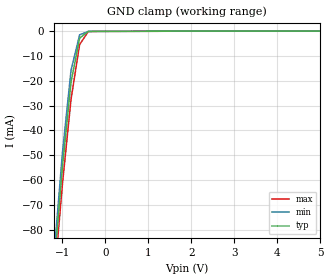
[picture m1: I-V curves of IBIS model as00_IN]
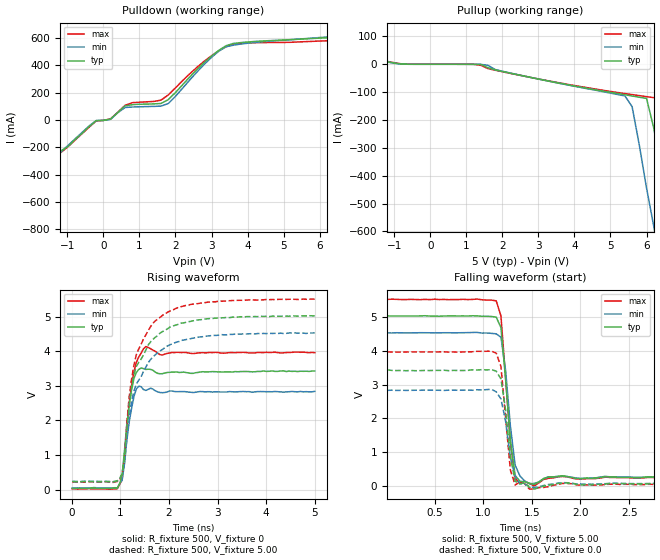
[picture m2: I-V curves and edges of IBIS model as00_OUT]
| TEXas INSTRUMENTS INCORPORATED
| Standard Linear and Logic Group
| IBIS Model of SN74as00
| QUADRUPLE 2-INPUT POSITIVE-NAND GATES
| SOIC 14-pin (D), SOP 14-pin (NS), PDIP 14-pin (N) packages
[IBIS Ver]   3.2
[Comment Char]  |_char
[File Name]   sn74as00.ibs
[File Rev]   3.1 I_die
[Date]   Sept. 29, 2004
[Source]   File originated at Texas Instruments, Inc.
[Notes]   The following is an IBIS list for the as00.
   - FILE REV HISTORY
   - 3.1 Re-Release IBIS file on 10/06/04
   - Power clamp data deleted as there is no power-clamp diode.
   - All test data contained in this file are derived from
   actual measurements.
   - File created by Nobuhisa Ohtsubo, SLL Product Engineering.
[Disclaimer] Property of Texas Instruments Incorporated.  Unauthorized
   reproduction and/or distribution is strictly prohibited.
   This product is protected under copyright law.
   Created 2000, (C) Copyright 2000, Texas Instruments Inc.,
   All Rights Reserved.
   UNLESS THERE IS A SIGNED, WRITTEN AGREEMENT TO THE
   CONTRARY, TEXas INSTRUMENTS () IS PROVIDING THE IBIS
   MODELS  AND WITHOUT ANY WARRANTY, EXPRESSED OR
   IMPLIED.  TI assumes no liability for:
   1) the accuracy of the IBIS models provided to your
   company;
   2) the proper functioning of these IBIS Models in your
   design or for any resulting applications; or
   3) infringement of patents, copyrights or intellectual
   property rights resulting from your use of these IBIS
   models.
   TI provides IBIS Models as a service to our customers.
   You and your company shall not distribute, sell or give
   these models to anyone else without prior written
   permission from TI.
   TI reserves the right to make changes to our products or
   to discontinue any semiconductor product or service
   without notice, and advises our customers to obtain the
   latest version of relevant information to verify, before
   placing orders, that the information being relied on is
   current.
   Please be aware that your receipt and use of the IBIS
   information provided shall serve as acceptance of these
   terms and conditions.  If you do not accept these terms,
   you should return or destroy the IBIS models and any
   other accompanying information immediately.
|   Component as00_D
[Component]   as00_D
[Manufacturer]  Texas Instruments, Inc.
[Package]
|   typ   min   max
R_pkg   0.031   0.028   0.034
L_pkg   3.109nH   2.462nH   3.889nH
C_pkg   0.473pF   0.363pF   0.628pF
[Pin]   signal_name   model_name   R_pin   L_pin   C_pin
1   1A   as00_IN   0.033   3.854nH   0.622pF
2   1B   as00_IN   0.032   3.188nH   0.473pF
3   1Y   as00_OUT   0.028   2.462nH   0.377pF
4   2A   as00_IN   0.031   2.596nH   0.363pF
5   2B   as00_IN   0.028   2.521nH   0.372pF
6   2Y   as00_OUT   0.034   3.250nH   0.476pF
7   GND   GND   0.034   3.889nH   0.628pF
8   3Y   as00_OUT   0.034   3.889nH   0.628pF
9   3A   as00_IN   0.034   3.250nH   0.476pF
10   3B   as00_IN   0.028   2.521nH   0.372pF
11   4Y   as00_OUT   0.031   2.596nH   0.364pF
12   4A   as00_IN   0.028   2.462nH   0.377pF
13   4B   as00_IN   0.032   3.188nH   0.473pF
14   VCC   POWER   0.033   3.854nH   0.622pF
|   Component as00_NS
[Component]   as00_NS
[Manufacturer]  Texas Instruments, Inc.
[Package]
|   typ   min   max
R_pkg   0.045   0.039   0.054
L_pkg   3.796nH   2.561nH   4.952nH
C_pkg   0.528pF   0.288pF   0.710pF
[Pin]   signal_name   model_name   R_pin   L_pin   C_pin
1   1A   as00_IN   0.047   4.867nH   0.706pF
2   1B   as00_IN   0.051   4.083nH   0.592pF
3   1Y   as00_OUT   0.041   2.915nH   0.376pF
4   2A   as00_IN   0.039   2.561nH   0.288pF
5   2B   as00_IN   0.041   3.101nH   0.430pF
6   2Y   as00_OUT   0.047   4.047nH   0.589pF
7   GND   GND   0.051   4.909nH   0.700pF
8   3Y   as00_OUT   0.045   4.784nH   0.694pF
9   3A   as00_IN   0.054   4.176nH   0.597pF
10   3B   as00_IN   0.039   3.287nH   0.449pF
11   4Y   as00_OUT   0.039   2.586nH   0.294pF
12   4A   as00_IN   0.040   2.802nH   0.371pF
13   4B   as00_IN   0.049   4.080nH   0.593pF
14   VCC   POWER   0.052   4.952nH   0.710pF
|   Component as00_N
[Component]   as00_N
[Manufacturer]   Texas Instruments, Inc.
[Package]
|   typ   min   max
R_pkg   4.500e-02   3.700e-02   6.300e-02
L_pkg   5.407e-09   3.922e-09   6.942e-09
C_pkg   3.890e-13   2.050e-13   6.040e-13
[Pin]   signal_name   model_name   R_pin   L_pin   C_pin
1   1A   as00_IN   6.300e-02   6.942e-09   6.040e-13
2   1B   as00_IN   3.700e-02   6.200e-09   4.060e-13
3   1Y   as00_OUT   4.200e-02   4.389e-09   3.220e-13
4   2A   as00_IN   3.800e-02   3.922e-09   2.050e-13
5   2B   as00_IN   3.900e-02   4.301e-09   2.980e-13
6   2Y   as00_OUT   3.800e-02   5.329e-09   3.560e-13
7   GND   GND   5.300e-02   6.510e-09   5.440e-13
8   3Y   as00_OUT   5.300e-02   6.437e-09   5.390e-13
9   3A   as00_IN   3.900e-02   5.352e-09   3.470e-13
10   3B   as00_IN   4.200e-02   4.473e-09   2.970e-13
11   4Y   as00_OUT   4.400e-02   4.326e-09   2.250e-13
12   4A   as00_IN   4.200e-02   4.295e-09   2.800e-13
13   4B   as00_IN   4.200e-02   6.318e-09   4.180e-13
14   VCC   POWER   6.100e-02   6.900e-09   6.030e-13
| Models and submodels in the file (2): as00_IN (Input), as00_OUT (Output)
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|   Model as00_IN
[Model]   as00_IN
Model_type  Input
Polarity   Non-Inverting
Vinl = 0.8
Vinh = 2.0
| variable   typ   min   max
C_comp   1.33pf   1.00pf   1.66pf
[Temperature Range]   25   0   70
[Voltage Range]   5.0   4.5   5.5
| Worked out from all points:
|   GND clamp passes 1 mA (typ) near -0.46 V on its own axis
[GND Clamp]
|   Voltage   I(typ)   I(min)   I(max)
-5V       -1.126A    -1.168A    -1.087A
-1.2V     -96.27mA   -91.36mA   -102.1mA
-1V       -54.78mA   -49.12mA   -61.66mA
-800mV    -20.6mA    -15.82mA   -27.49mA
-600mV    -2.839mA   -1.5mA     -5.406mA
-400mV    -139.7uA   -123.8uA   -215.7uA
5V        170pA      183.6pA    226.4pA
|   Model as00_OUT
[Model]   as00_OUT
Model_type  Output
Polarity   Inverting
Enable   Active-Low
Vmeas = 1.3v
Cref = 0pf
| variable   typ   min   max
C_comp   5.8pf   4.35pf   7.25pf
[Temperature Range]   25   0   70
[Voltage Range]   5.0   4.5   5.5
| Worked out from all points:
|   slope of the pulldown table from 0 to 0.75 V, typ, clamps not added: 6.65 ohm
|   slope of the pullup table from 0 to 0.75 V, typ, clamps not added: 22.6 kohm
|   rising waveform, R_fixture 500, V_fixture 0: 20-80 % time 160ps typ, 152ps min, 176ps max; typ from 0.031 V to 3.43 V
|   falling waveform, R_fixture 500, V_fixture 5.00: 20-80 % time 84.4ps typ, 89.7ps min, 82.1ps max; typ from 5.05 V to 0.24 V
|   rising waveform, R_fixture 500, V_fixture 5.00: 20-80 % time 433ps typ, 469ps min, 411ps max; typ from 0.23 V to 5.02 V
|   falling waveform, R_fixture 500, V_fixture 0.0: 20-80 % time 84.8ps typ, 94.7ps min, 74.7ps max; typ from 3.44 V to 0.043 V
[Pulldown]
|   Voltage   I(typ)   I(min)   I(max)
-5V       -2.513A    -2.408A    -2.451A
-2.2V     -859.8mA   -830.5mA   -846.9mA
-2V       -741.7mA   -717.8mA   -732.3mA
-1.6V     -517mA     -521.7mA   -510.6mA
-1.2V     -227.4mA   -239.2mA   -241.5mA
-200mV    -4.196mA   -3.233mA   -5.919mA
200mV     7.396mA    5.741mA    9.506mA
600mV     103.7mA    92.22mA    108mA
1.8V      149.8mA    121.4mA    184.6mA
2.8V      422.2mA    408.7mA    431.4mA
3.4V      544.1mA    536.6mA    537.1mA
10V       655.6mA    682.5mA    620.9mA
[Pullup]
|   Voltage   II(typ)   I(min)   I(max)
-5V       115.7mA    126.5mA    99.43mA
-1V       4.25mA     3.482mA    5.401mA
1.6V      -12.64mA   -3.784mA   -15.45mA
5.4V      -109.5mA   -113.6mA   -105.2mA
5.6V      -113.9mA   -152.3mA   -108.8mA
6V        -122.7mA   -444.5mA   -116.2mA
6.2V      -228.6mA   -581.2mA   -119.9mA
6.4V      -370.2mA   -720.9mA   -123.6mA
6.6V      -518.5mA   -860.6mA   -180.5mA
6.8V      -643.6mA   -1A        -305.7mA
7.2V      -913.2mA   -1.28A     -569.1mA
10V       -2.801A    -3.236A    -2.375A
[Ramp]
| variable   typ   min   max
dV/dt_r   1.940E+00/1.520E-09  1.600E+00/1.490E-09  2.290E+00/1.710E-09
dV/dt_f   2.880E+00/8.100E-10  2.580E+00/8.400E-10  3.180E+00/7.800E-10
R_load = 500
[Rising Waveform]
R_fixture = 500
V_fixture = 0
C_fixture = 0pf
L_fixture = 0nH
|   Time   V(typ)   V(min)   V(max)
9.766ps   31.22mV    44.19mV    19.5mV
937.5ps   42.63mV    43.72mV    22.32mV
1.035ns   414mV      269mV      280.4mV
1.133ns   1.898V     1.425V     1.782V
1.182ns   2.428V     1.956V     2.505V
1.279ns   3.21V      2.688V     3.405V
1.377ns   3.47V      2.987V     3.827V
1.523ns   3.47V      2.865V     4.131V
1.865ns   3.348V     2.798V     3.888V
5ns       3.427V     2.838V     3.954V
[Falling Waveform]
R_fixture = 500
V_fixture = 5.00
V_fixture_min = 4.50
V_fixture_max = 5.50
C_fixture = 0pf
L_fixture = 0nH
|   Time   V(typ)   V(min)   V(max)
9.766ps   5.047V     4.543V     5.538V
1.133ns   5.012V     4.513V     5.495V
1.182ns   4.699V     4.415V     5.045V
1.23ns    3.153V     3.418V     3.192V
1.279ns   1.337V     1.77V      1.285V
1.328ns   299.7mV    603.1mV    200.4mV
1.377ns   127mV      286.4mV    77mV
1.475ns   69.03mV    50.13mV    59.5mV
1.816ns   289.3mV    283.1mV    269.2mV
5ns       239.7mV    246.5mV    230mV
[Rising Waveform]
R_fixture = 500
V_fixture = 5.00
V_fixture_min = 4.50
V_fixture_max = 5.50
C_fixture = 0pf
L_fixture = 0nH
|   Time   V(typ)   V(min)   V(max)
9.766ps   230.4mV    235.6mV    207.8mV
986.3ps   312.9mV    316.1mV    291.2mV
1.035ns   455.4mV    443.7mV    442.8mV
1.084ns   919.7mV    786.5mV    922.2mV
1.182ns   2.49V      2.073V     2.695V
1.328ns   3.554V     3.047V     3.898V
1.621ns   4.268V     3.757V     4.706V
1.865ns   4.563V     4.048V     5.033V
3.066ns   4.963V     4.481V     5.443V
5ns       5.018V     4.528V     5.502V
[Falling Waveform]
R_fixture = 500
V_fixture = 0.0
V_fixture_min = 0.0
V_fixture_max = 0.0
C_fixture = 0pf
L_fixture = 0nH
|   Time   V(typ)   V(min)   V(max)
9.766ps   3.443V     2.831V     3.977V
1.133ns   3.403V     2.788V     3.94V
1.182ns   3.172V     2.578V     3.543V
1.23ns    2.246V     1.909V     2.008V
1.279ns   857.3mV    823mV      457.2mV
1.328ns   127.9mV    280mV      16.06mV
1.377ns   43.25mV    57.32mV    104mV
1.475ns   -55.65mV   -31.59mV   -108.6mV
1.816ns   75.6mV     86.85mV    64.19mV
5ns       42.78mV    51.22mV    17.16mV
